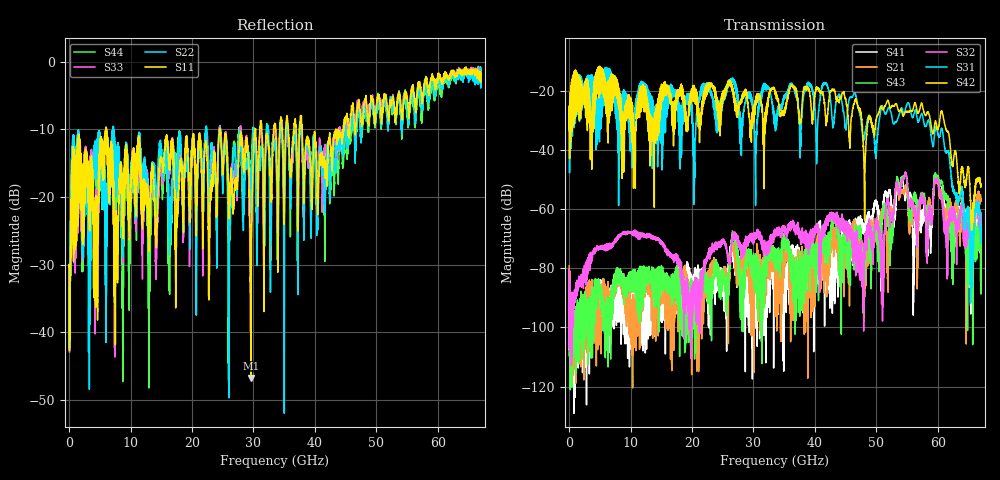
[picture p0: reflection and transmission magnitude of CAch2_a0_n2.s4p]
!Agilent Technologies,N5247A,US51170199,A.09.90.13
!Agilent N5247A: A.09.90.13
!Date: Thursday, October 18, 2018 09:22:54
!Correction: S11(Full 4 Port(1,2,3,4))
!S12(Full 4 Port(1,2,3,4))
!S13(Full 4 Port(1,2,3,4))
!S14(Full 4 Port(1,2,3,4))
!S21(Full 4 Port(1,2,3,4))
!S22(Full 4 Port(1,2,3,4))
!S23(Full 4 Port(1,2,3,4))
!S24(Full 4 Port(1,2,3,4))
!S31(Full 4 Port(1,2,3,4))
!S32(Full 4 Port(1,2,3,4))
!S33(Full 4 Port(1,2,3,4))
!S34(Full 4 Port(1,2,3,4))
!S41(Full 4 Port(1,2,3,4))
!S42(Full 4 Port(1,2,3,4))
!S43(Full 4 Port(1,2,3,4))
!S44(Full 4 Port(1,2,3,4))
!S4P File: Measurements: <S11,S12,S13,S14>,
!<S21,S22,S23,S24>,
!<S31,S32,S33,S34>,
!<S41,S42,S43,S44>:
# Hz S  dB  R 50
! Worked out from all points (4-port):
!   6701 points, 10 MHz to 67 GHz, reference 50 ohm
!   strongest paths, dB at 10 MHz, 16.76 GHz, 33.51 GHz, 50.25 GHz, 67 GHz:
!     S42: -32.9, -25.8, -19.8, -27.9, -52.1
!     S31: -33.4, -22.3, -30.0, -33.2, -67.7
!     S32: -80.5, -75.5, -69.0, -66.0, -63.9
!     S43: -87.4, -82.6, -75.3, -69.8, -70.4
!     S21: -79.2, -95.1, -79.8, -68.5, -57.3
!     S41: -80.6, -86.6, -81.0, -59.4, -68.6
!   lowest |S11| = -46.7 dB at 29.59 GHz (marker M1), VSWR 1.01, Z = 50.3 - j0.329 ohm
!   |S11| at or under -10 dB: start of sweep to 5.978 GHz; 6.102 GHz to 24.48 GHz (18.38 GHz wide, 120 % of centre); 24.51 GHz to 30.25 GHz (5.737 GHz wide, 21 % of centre)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
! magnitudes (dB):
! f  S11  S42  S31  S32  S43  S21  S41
! 10 MHz  -30.4  -32.9  -33.4  -80.5  -87.4  -79.2  -80.6
! 5.989 GHz  -9.8  -17.2  -12.2  -73.4  -104.5  -87.3  -88.6
! 20.35 GHz  -11.4  -23.1  -41.5  -89.4  -96.0  -91.4  -83.6
! 29.59 GHz  -46.7  -32.7  -21.6  -69.6  -74.4  -85.7  -91.6
! 47.64 GHz  -8.7  -30.5  -33.4  -81.4  -74.3  -76.7  -64.9
! 55.18 GHz  -6.6  -26.9  -24.0  -55.2  -57.8  -61.8  -54.9
! 67 GHz  -3.1  -52.1  -67.7  -63.9  -70.4  -57.3  -68.6
